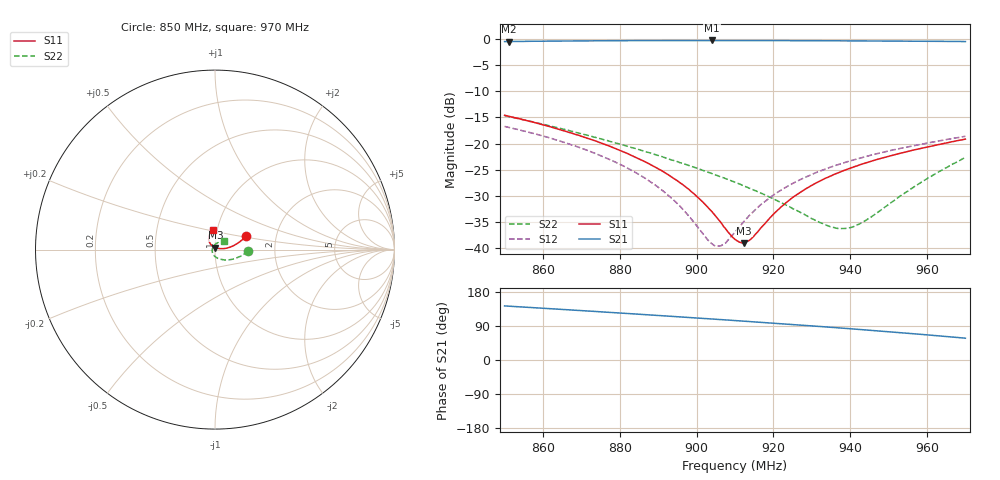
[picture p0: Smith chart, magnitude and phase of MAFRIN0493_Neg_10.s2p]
!Part Number:  MAFRIN0493
!Name:  MC
!Comments:  1
!Thu 09/Dec/2004  3:51:09 PM
!Temperature:  -10
# MHZ  S  DB  R  50
!Freq  S11(dB)  S11(ang)  S21(dB)  S21(ang)  S12(dB)  S12(ang)  S22(dB)  S22(ang)
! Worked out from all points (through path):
!   201 points, 850 MHz to 970 MHz, reference 50 ohm
!   highest |S21| = -0.22 dB at 904 MHz (marker M1); lowest = -0.4 dB at 851.2 MHz (marker M2)
!   group delay of S21, straight-line fit = 1.94 ns
!   lowest |S11| = -39.1 dB at 912.4 MHz (marker M3), VSWR 1.02, Z = 50.3 + j1.08 ohm
!   |S11| at or under -10 dB: start of sweep to end of sweep
!   |S22| runs from -36.3 to -14.7 dB; largest |S21 - S12| = 1.1
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850  -14.58 23.6  -0.44 142.7  -16.72 103.7  -14.66 -2.8
851.2  -14.79 23.0  -0.44 142.0  -16.94 102.9  -14.86 -3.9
870.4  -18.71 13.5  -0.30 130.1  -21.02 92.3  -18.20 -23.4
881.2  -21.67 8.9  -0.26 123.2  -24.41 88.5  -20.36 -36.5
890.2  -24.94 6.7  -0.23 117.4  -28.50 88.9  -22.33 -48.8
894.4  -26.86 6.8  -0.24 114.6  -31.11 92.4  -23.34 -55.4
898  -28.80 7.9  -0.23 112.2  -33.93 99.5  -24.22 -61.2
904  -33.08 16.7  -0.22 108.2  -39.23 137.8  -25.76 -72.0
906.4  -35.23 24.6  -0.23 106.6  -39.60 165.5  -26.44 -76.5
907.6  -36.41 31.2  -0.23 105.8  -39.07 178.0  -26.75 -79.2
910  -38.41 49.6  -0.24 104.1  -37.00 -164.6  -27.45 -84.1
912.4  -39.09 75.7  -0.23 102.5  -34.90 -154.3  -28.15 -89.4
914.2  -38.32 93.7  -0.25 101.2  -33.51 -149.6  -28.71 -93.6
920.8  -33.01 123.3  -0.25 96.6  -29.49 -142.2  -30.91 -111.1
925  -30.36 128.1  -0.25 93.6  -27.67 -141.0  -32.49 -124.8
930.4  -27.85 129.0  -0.27 89.7  -25.81 -140.8  -34.54 -148.0
935.2  -26.15 127.6  -0.28 86.2  -24.47 -141.7  -36.07 -176.5
940  -24.74 125.3  -0.30 82.5  -23.32 -142.9  -36.15 149.7
944.2  -23.70 122.4  -0.30 79.2  -22.47 -144.1  -34.70 122.1
950.2  -22.43 117.8  -0.33 74.5  -21.42 -146.2  -31.59 93.3
959.8  -20.71 108.5  -0.37 66.6  -19.94 -149.4  -26.82 64.8
970  -19.16 97.2  -0.43 57.5  -18.61 -153.0  -22.71 43.8
